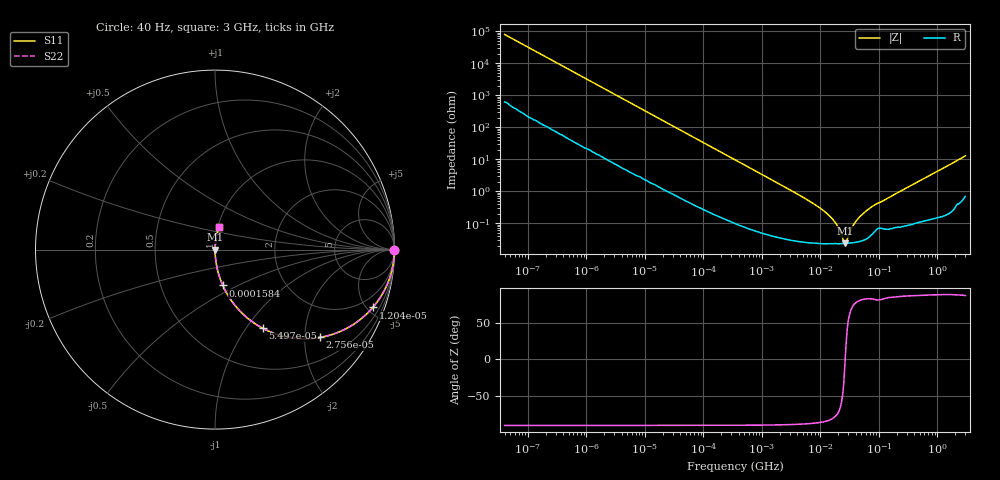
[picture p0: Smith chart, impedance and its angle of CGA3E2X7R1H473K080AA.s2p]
! S-parameter Generated by TDK Corporation
! Copyright(C) 2015 TDK Corporation.
! All Rights Reserved.
! TDK P/N: CGA3E2X7R1H473K080AA (Multilayer Ceramic Chip Capacitors)
! Property: C=47nF
! Size(LxWxT): 1.6x0.8x0.8mm, 0.063x0.031x0.031inches
! Model Type: s2p (Touchstone File Format Version 1.0)
! Frequency: DC=Yes Start=0.00004MHz Stop=3000MHz 396points Log-sweep
! Note: This model was converted from impedance.
! Model Generated on Jun. 23, 2015
! Hash(MD5):
! Port Assignments:
!  1 ---| |--- 2
! Applicable Conditions:
!  Temperature = 25 degC
!  DC Bias Voltage = 0 V
!  Small Signal Operation
! Terms and conditions regarding TDK Simulation Models
! (1)This simulation model is being provided solely for informational purposes. Please refer to the specifications of the products in terms of detailed characteristics of such products.
! (2)In no event shall TDK Corporation of any of its subsidiaries be liable for any loss or damage arising, directly or indirectly,
!  From any information contained in this simulation model, including, but not limited to loss or damages arising from any inaccuracies, omissions or errors in connection with such information.
! (3)Any and all copyrights on this simulation model are owned by TDK Corporation.
!  Duplication or redistribution of this simulation model without prior written permission from TDK Corporation is prohibited.
! (4)This simulation model is subject to any modification or change without any prior notice.
! (5)Neither TDK Corporation nor any of its subsidiaries shall make any warranty, express or implied,
!  Including but not limited to the correctness, implied warranties of merchantability and fitness for a particular purpose with respect to this simulation models.
! (6)The use of this simulation model shall be deemed to have consented to the terms and conditions hereof.
# MHz S MA R 50
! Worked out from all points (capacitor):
!   395 points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, 40 Hz to 3 GHz, reference 50 ohm
!   read as one part in series: C = 50 nF near 41.88 Hz
!   lowest |Z| = 23.4 mohm at 26.21 MHz (marker M1)
!   series resonance near 26.46 MHz, so ESL is about 720 pH
!   S11 on the Smith chart (normalised r, x): 40 Hz: open; 12.04 kHz: 1.04, -5.44; 27.56 kHz: 1.02, -2.38; 54.97 kHz: 1.01, -1.20; 158.4 kHz: 1.00, -0.42; 3 GHz: 1.01, +0.26
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4e-05  1 -0.1  0.00126 89.5  0.00126 89.5  1 -0.1
0.000834128  0.9995 -1.5  0.02576 88.1  0.02576 88.1  0.9995 -1.5
0.003809071  0.9925 -6.7  0.1161 83.0  0.1161 83.0  0.9925 -6.7
0.01203665  0.9364 -20.1  0.3443 69.5  0.3443 69.5  0.9364 -20.1
0.01739424  0.8807 -27.9  0.4673 61.7  0.4673 61.7  0.8807 -27.9
0.02756005  0.7634 -39.8  0.6404 49.8  0.6404 49.8  0.7634 -39.8
0.05496573  0.5125 -58.7  0.8548 30.8  0.8548 30.8  0.5125 -58.7
0.09119145  0.3399 -69.7  0.9377 19.9  0.9377 19.9  0.3399 -69.7
0.1584177  0.2045 -77.7  0.9771 11.8  0.9771 11.8  0.2045 -77.7
0.3464102  0.09564 -83.9  0.9944 5.5  0.9944 5.5  0.09564 -83.9
7.22376  0.004349 -86.6  0.9997 0.2  0.9997 0.2  0.004349 -86.6
11.98465  0.002264 -84.1  0.9998 0.1  0.9998 0.1  0.002264 -84.1
16.54008  0.001273 -79.5  0.9998 0.1  0.9998 0.1  0.001273 -79.5
20.81973  0.0006633 -69.8  0.9998 0.0  0.9998 0.0  0.0006633 -69.8
26.2067  0.0002336 -5.9  0.9998 0.0  0.9998 0.0  0.0002336 -5.9
27.44099  0.0002503 21.6  0.9998 -0.0  0.9998 -0.0  0.0002503 21.6
31.50375  0.0005083 61.6  0.9998 -0.0  0.9998 -0.0  0.0005083 61.6
36.16801  0.0008504 73.2  0.9998 -0.0  0.9998 -0.0  0.0008504 73.2
47.67047  0.001629 80.3  0.9997 -0.1  0.9997 -0.1  0.001629 80.3
79.08817  0.00347 81.9  0.9995 -0.2  0.9995 -0.2  0.00347 81.9
150.6385  0.006488 83.9  0.9993 -0.4  0.9993 -0.4  0.006488 83.9
3000  0.1264 79.7  0.9852 -7.2  0.9852 -7.2  0.1264 79.7
